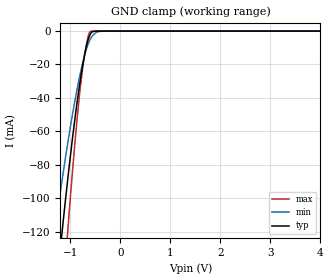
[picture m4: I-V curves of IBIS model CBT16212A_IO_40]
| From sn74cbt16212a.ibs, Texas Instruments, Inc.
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[Model]   CBT16212A_IO_40
Model_type  Terminator
| variable   typ   min   max
C_comp   5.31pF   4.39pF   6.77pF
| C_tri-state   5.31pF   4.39pF   6.77pF
[Temperature Range]   40   100   -40
| Ambient temperature   25   85   -40
[Voltage range]   4   4   4
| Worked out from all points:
|   GND clamp passes 1 mA (typ) near -0.58 V on its own axis
[GND Clamp]
| CBT16212A_IO_40
|   Voltage   I(typ)   I(min)   I(max)
-4V       -1.21A     -907.6mA   -1.656A
-1.335V   -170.7mA   -125.3mA   -238.1mA
-1.295V   -158.3mA   -116.4mA   -220.4mA
-1.18V    -123.9mA   -91.93mA   -170.8mA
-1.075V   -94.34mA   -71.02mA   -127.9mA
-1.04V    -84.94mA   -64.41mA   -114.2mA
-890mV    -47.82mA   -38.43mA   -60.13mA
-775mV    -24mA      -21.58mA   -26.74mA
-670mV    -7.818mA   -9.77mA    -6.233mA
-590mV    -1.22mA    -4.149mA   -82.86uA
-340mV    -466.3nA   -31.67uA   -4.233nA
4V        75.6pA     3.282nA    35.34pA
